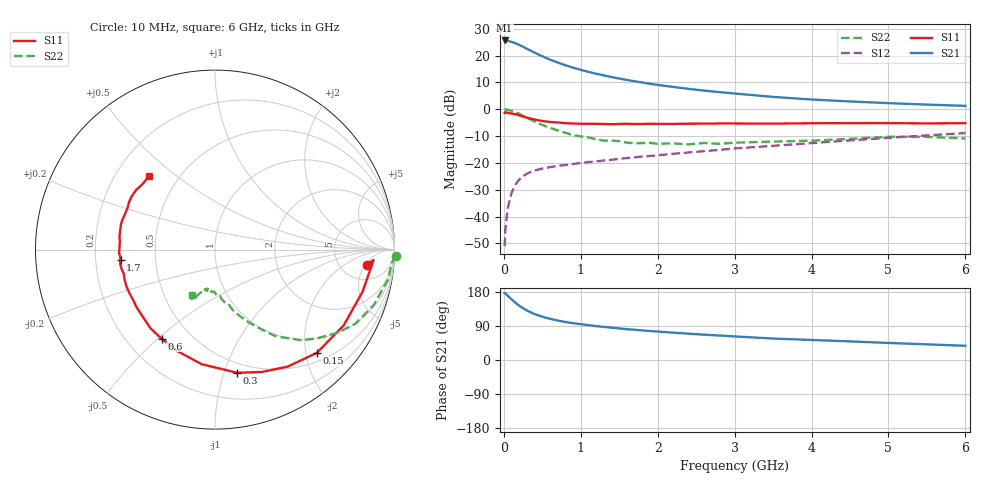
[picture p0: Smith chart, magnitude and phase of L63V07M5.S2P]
!  INFINEON TECHNOLOGIES Small Signal Semiconductors
! BFR380L3 , Si-NPN RF-Transistor in TSLP-3-1
!  Vce=3 V,  Ic=7.5 mA
! Common Emitter S-Parameters:  07. March 2005
#  GHz  S  MA  R  50
! f  S11  S21  S12  S22
! GHz  Mag  Ang  Mag  Ang  Mag  Ang  Mag  Ang
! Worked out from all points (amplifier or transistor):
!   36 points, 10 MHz to 6 GHz, reference 50 ohm
!   highest |S21| = 25.6 dB at 10 MHz (marker M1)
!   |S21| within 3 dB of that: start of sweep to 292.3 MHz
!   unconditionally stable (mu >= 1): 2.251 GHz to 4.72 GHz
!   at 250 MHz: K = 0.22, MSG = 24.1 dB, |S12| = -25.0 dB
!   at 1.4 GHz: K = 0.85, MSG = 15.4 dB, |S12| = -18.8 dB
!   at 6 GHz: K = 0.95, MSG = 5.1 dB, |S12| = -8.9 dB
!   S11 on the Smith chart (normalised r, x): 10 MHz: 9, -6; 150 MHz: 0.67, -2.22; 300 MHz: 0.41, -1.11; 600 MHz: 0.34, -0.51; 1.7 GHz: 0.31, -0.05; 6 GHz: 0.34, +0.40
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0.01  0.8529 -5.6  19.14 176.2  0.0028 85.8  1.009 -2.0
0.02  0.8856 -3.7  19.08 176.1  0.0057 93.9  0.9883 -4.1
0.05  0.8551 -15.9  18.83 169.7  0.0141 82.0  0.9779 -9.8
0.1  0.8322 -30.5  18.05 160.2  0.0276 74.4  0.9377 -19.1
0.15  0.8081 -45.4  17.07 151.1  0.0394 68.0  0.8852 -27.8
0.2  0.7678 -58.1  15.82 143.2  0.0487 62.9  0.8224 -34.4
0.25  0.7299 -69.1  14.6 136.7  0.0564 58.4  0.7532 -41.0
0.3  0.6973 -79.8  13.37 130.6  0.0629 54.8  0.6977 -46.4
0.4  0.6426 -96.7  11.35 121.2  0.0722 49.6  0.5891 -55.0
0.5  0.6039 -109.9  9.722 114.3  0.0782 47.2  0.5092 -60.1
0.6  0.5787 -121.0  8.403 108.6  0.0831 45.4  0.4498 -64.9
0.7  0.5671 -129.3  7.416 104.3  0.0881 45.3  0.4013 -68.9
0.8  0.5492 -137.2  6.615 100.4  0.0912 44.9  0.3635 -72.7
1.1  0.535 -153.3  4.973 91.8  0.1035 46.5  0.2973 -79.8
1.4  0.5252 -164.7  3.973 85.4  0.1142 48.7  0.26 -84.9
1.7  0.5287 -173.6  3.317 79.8  0.1267 50.9  0.2322 -91.2
2.2  0.5318 175.5  2.606 72.1  0.1475 54.4  0.2306 -96.5
2.8  0.5423 164.8  2.086 64.6  0.1746 57.6  0.2268 -104.1
3.5  0.5391 155.1  1.697 56.6  0.2078 58.7  0.2493 -107.8
4.5  0.5508 147.4  1.396 49.1  0.2627 60.7  0.2801 -111.5
5.5  0.5442 138.0  1.22 41.3  0.3248 59.7  0.3046 -114.8
6  0.55 132.1  1.156 37.5  0.3594 58.3  0.2852 -116.8
